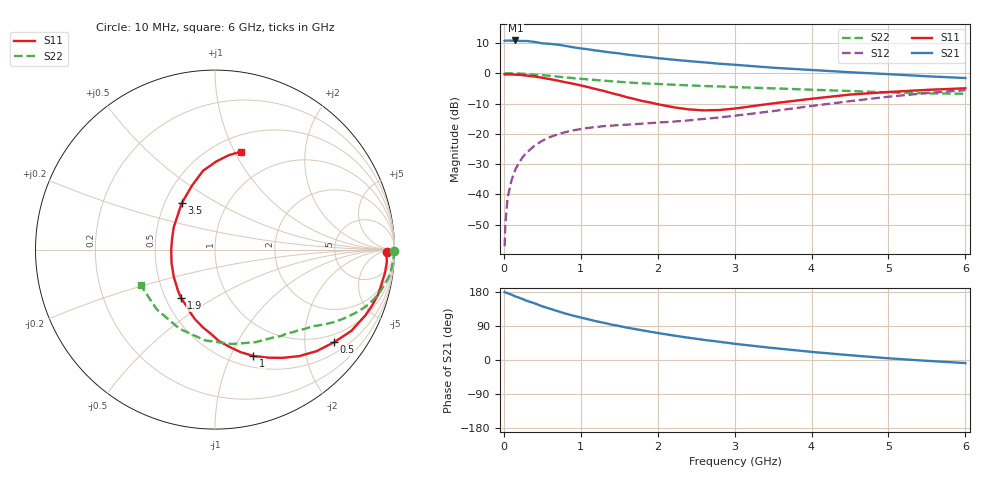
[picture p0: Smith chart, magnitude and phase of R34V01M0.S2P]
! SIEMENS Small Signal Semiconductors
! BFR181
! Si NPN RF Bipolar Junction Transistor in SOT23
! VCE = 4 V  IC = 1 mA
! Common Emitter S-Parameters:  May  1996
# GHz  S  MA  R  50
!  f  S11  S21  S12  S22
! GHz  MAG  ANG  MAG  ANG  MAG  ANG  MAG  ANG
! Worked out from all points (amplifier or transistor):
!   36 points, 10 MHz to 6 GHz, reference 50 ohm
!   highest |S21| = 10.8 dB at 150 MHz (marker M1)
!   |S21| within 3 dB of that: start of sweep to 1.115 GHz
!   unconditionally stable (mu >= 1): 2.033 GHz to 3.672 GHz
!   at 250 MHz: K = 0.15, MSG = 19.1 dB, |S12| = -27.5 dB
!   at 1.4 GHz: K = 0.77, MSG = 12.0 dB, |S12| = -17.3 dB
!   at 6 GHz: K = 0.87, MSG = 2.0 dB, |S12| = -5.6 dB
!   lowest NFmin = 1.30 dB at 450 MHz
!   S11 on the Smith chart (normalised r, x): 10 MHz: 46, -14; 500 MHz: 0.77, -2.73; 1 GHz: 0.62, -1.22; 1.9 GHz: 0.60, -0.36; 3.5 GHz: 0.61, +0.35; 6 GHz: 0.66, +1.06
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0.01  0.9607 -0.7  3.427 179.5  0.0014 91.3  0.9997 -0.4
0.02  0.955 -1.5  3.463 178.4  0.0033 89.1  0.9933 -0.8
0.05  0.9599 -3.9  3.466 176.1  0.009 88.4  0.9971 -1.9
0.1  0.956 -7.8  3.437 172.6  0.0172 83.6  0.9943 -3.7
0.15  0.9475 -11.7  3.477 167.7  0.0258 81.0  0.9899 -5.7
0.3  0.9141 -23.7  3.406 156.1  0.0494 75.4  0.969 -10.9
0.4  0.8844 -30.8  3.286 149.6  0.0641 70.4  0.9503 -14.2
0.5  0.841 -37.8  3.12 141.7  0.0769 66.1  0.9293 -17.1
0.7  0.7563 -51.7  2.965 128.8  0.0979 58.9  0.8793 -22.4
0.8  0.7099 -58.2  2.829 122.6  0.1068 55.5  0.8547 -24.6
1  0.6301 -70.1  2.571 112.1  0.12 50.9  0.8108 -28.4
1.1  0.5889 -76.0  2.478 107.3  0.1255 49.0  0.7906 -30.1
1.4  0.4691 -92.9  2.19 93.5  0.1366 45.2  0.7379 -34.5
1.6  0.4023 -106.3  2.033 85.3  0.1419 44.2  0.7079 -36.8
1.9  0.3302 -124.8  1.845 74.8  0.1502 44.4  0.6744 -40.4
2.2  0.2753 -146.5  1.676 64.8  0.1589 45.6  0.6465 -44.1
2.6  0.244 -179.9  1.514 53.2  0.1762 48.4  0.6152 -49.3
3  0.2613 151.8  1.381 42.8  0.1988 50.6  0.59 -55.8
3.5  0.3181 125.7  1.234 31.6  0.2375 51.7  0.5633 -66.3
4.5  0.4444 98.6  1.039 12.6  0.3466 47.5  0.5089 -96.2
5.5  0.5316 81.7  0.891 -2.2  0.4705 35.0  0.4652 -134.2
6  0.5649 75.1  0.834 -8.1  0.5259 27.2  0.4589 -154.5
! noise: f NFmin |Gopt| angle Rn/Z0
0.45  1.3  0.7  18  0.5
0.9  1.4  0.6  39  0.52
1.8  1.85  0.4  81  0.47
